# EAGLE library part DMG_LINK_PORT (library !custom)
DMG Link port; used to communicate with other Gameboys.
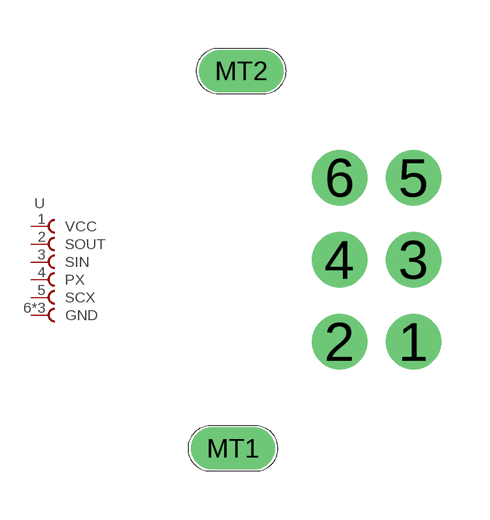
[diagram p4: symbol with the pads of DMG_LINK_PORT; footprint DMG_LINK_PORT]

Designator prefix -

## DMG_LINK_PORT  [DMG_LINK_PORT]
1  VCC  pas
2  SOUT  pas
3  SIN  pas
4  PX  pas
5  SCX  pas
6  GND  pas
MT1  GND  pas
MT2  GND  pas

## Footprint DMG_LINK_PORT (pad centres in mm)
drill 1.143 pad 1.422: 1 7.366,-2.54; 2 5.08,-2.54; 3 7.366,0; 4 5.08,0; 5 7.366,2.54; 6 5.08,2.54
drill 0.8 long: MT1 1.778,-5.842; MT2 2.032,5.842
